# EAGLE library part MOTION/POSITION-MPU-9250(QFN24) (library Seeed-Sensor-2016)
314990005
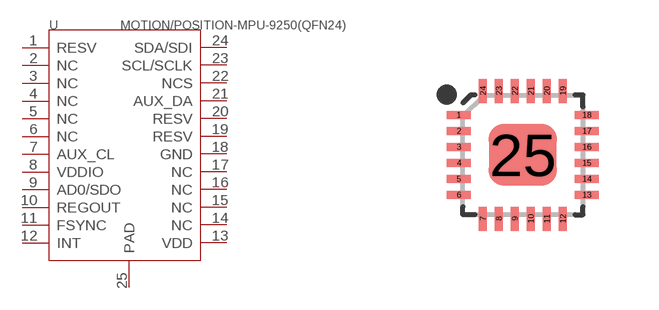
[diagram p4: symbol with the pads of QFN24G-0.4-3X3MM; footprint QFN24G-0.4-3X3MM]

Designator prefix U

## MOTION/POSITION-MPU-9250(QFN24) (MPN: MPU-9250; VALUE: MPU-9250)  [QFN24G-0.4-3X3MM]
1  RESV
2  NC
3  NC
4  NC
5  NC
6  NC
7  AUX_CL
8  VDDIO
9  AD0/SDO
10  REGOUT
11  FSYNC
12  INT
13  VDD
14  NC
15  NC
16  NC
17  NC
18  GND
19  RESV
20  RESV
21  AUX_DA
22  NCS
23  SCL/SCLK
24  SDA/SDI
25  PAD

## Footprint QFN24G-0.4-3X3MM (pad centres in mm)
smd 0.6 x 0.2: 1 -1.6,1; 2 -1.6,0.6; 3 -1.6,0.2; 4 -1.6,-0.2; 5 -1.6,-0.6; 6 -1.6,-1; 13 1.6,-1; 14 1.6,-0.6; 15 1.6,-0.2; 16 1.6,0.2; 17 1.6,0.6; 18 1.6,1
smd 0.2 x 0.6: 7 -1,-1.6; 8 -0.6,-1.6; 9 -0.2,-1.6; 10 0.2,-1.6; 11 0.6,-1.6; 12 1,-1.6; 19 1,1.6; 20 0.6,1.6; 21 0.2,1.6; 22 -0.2,1.6; 23 -0.6,1.6; 24 -1,1.6
smd 1.7 x 1.54: 25 0,0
